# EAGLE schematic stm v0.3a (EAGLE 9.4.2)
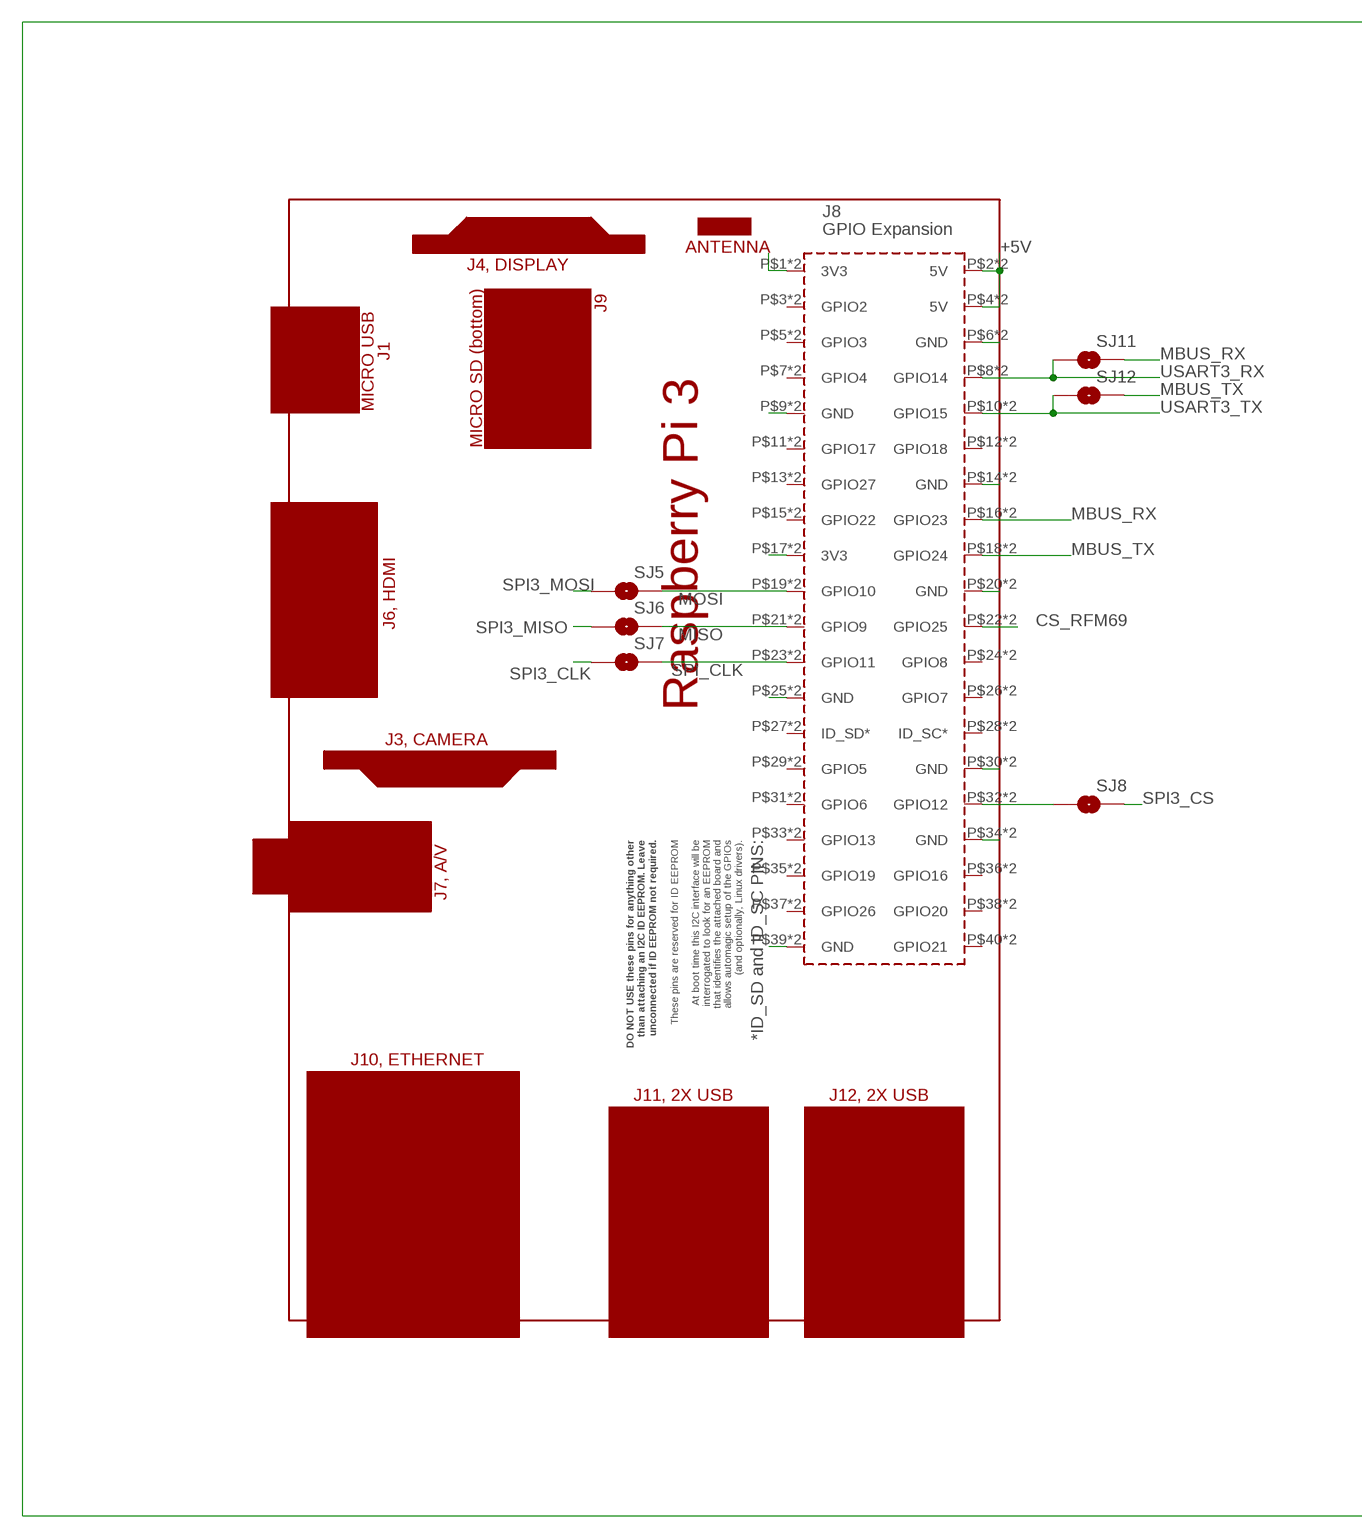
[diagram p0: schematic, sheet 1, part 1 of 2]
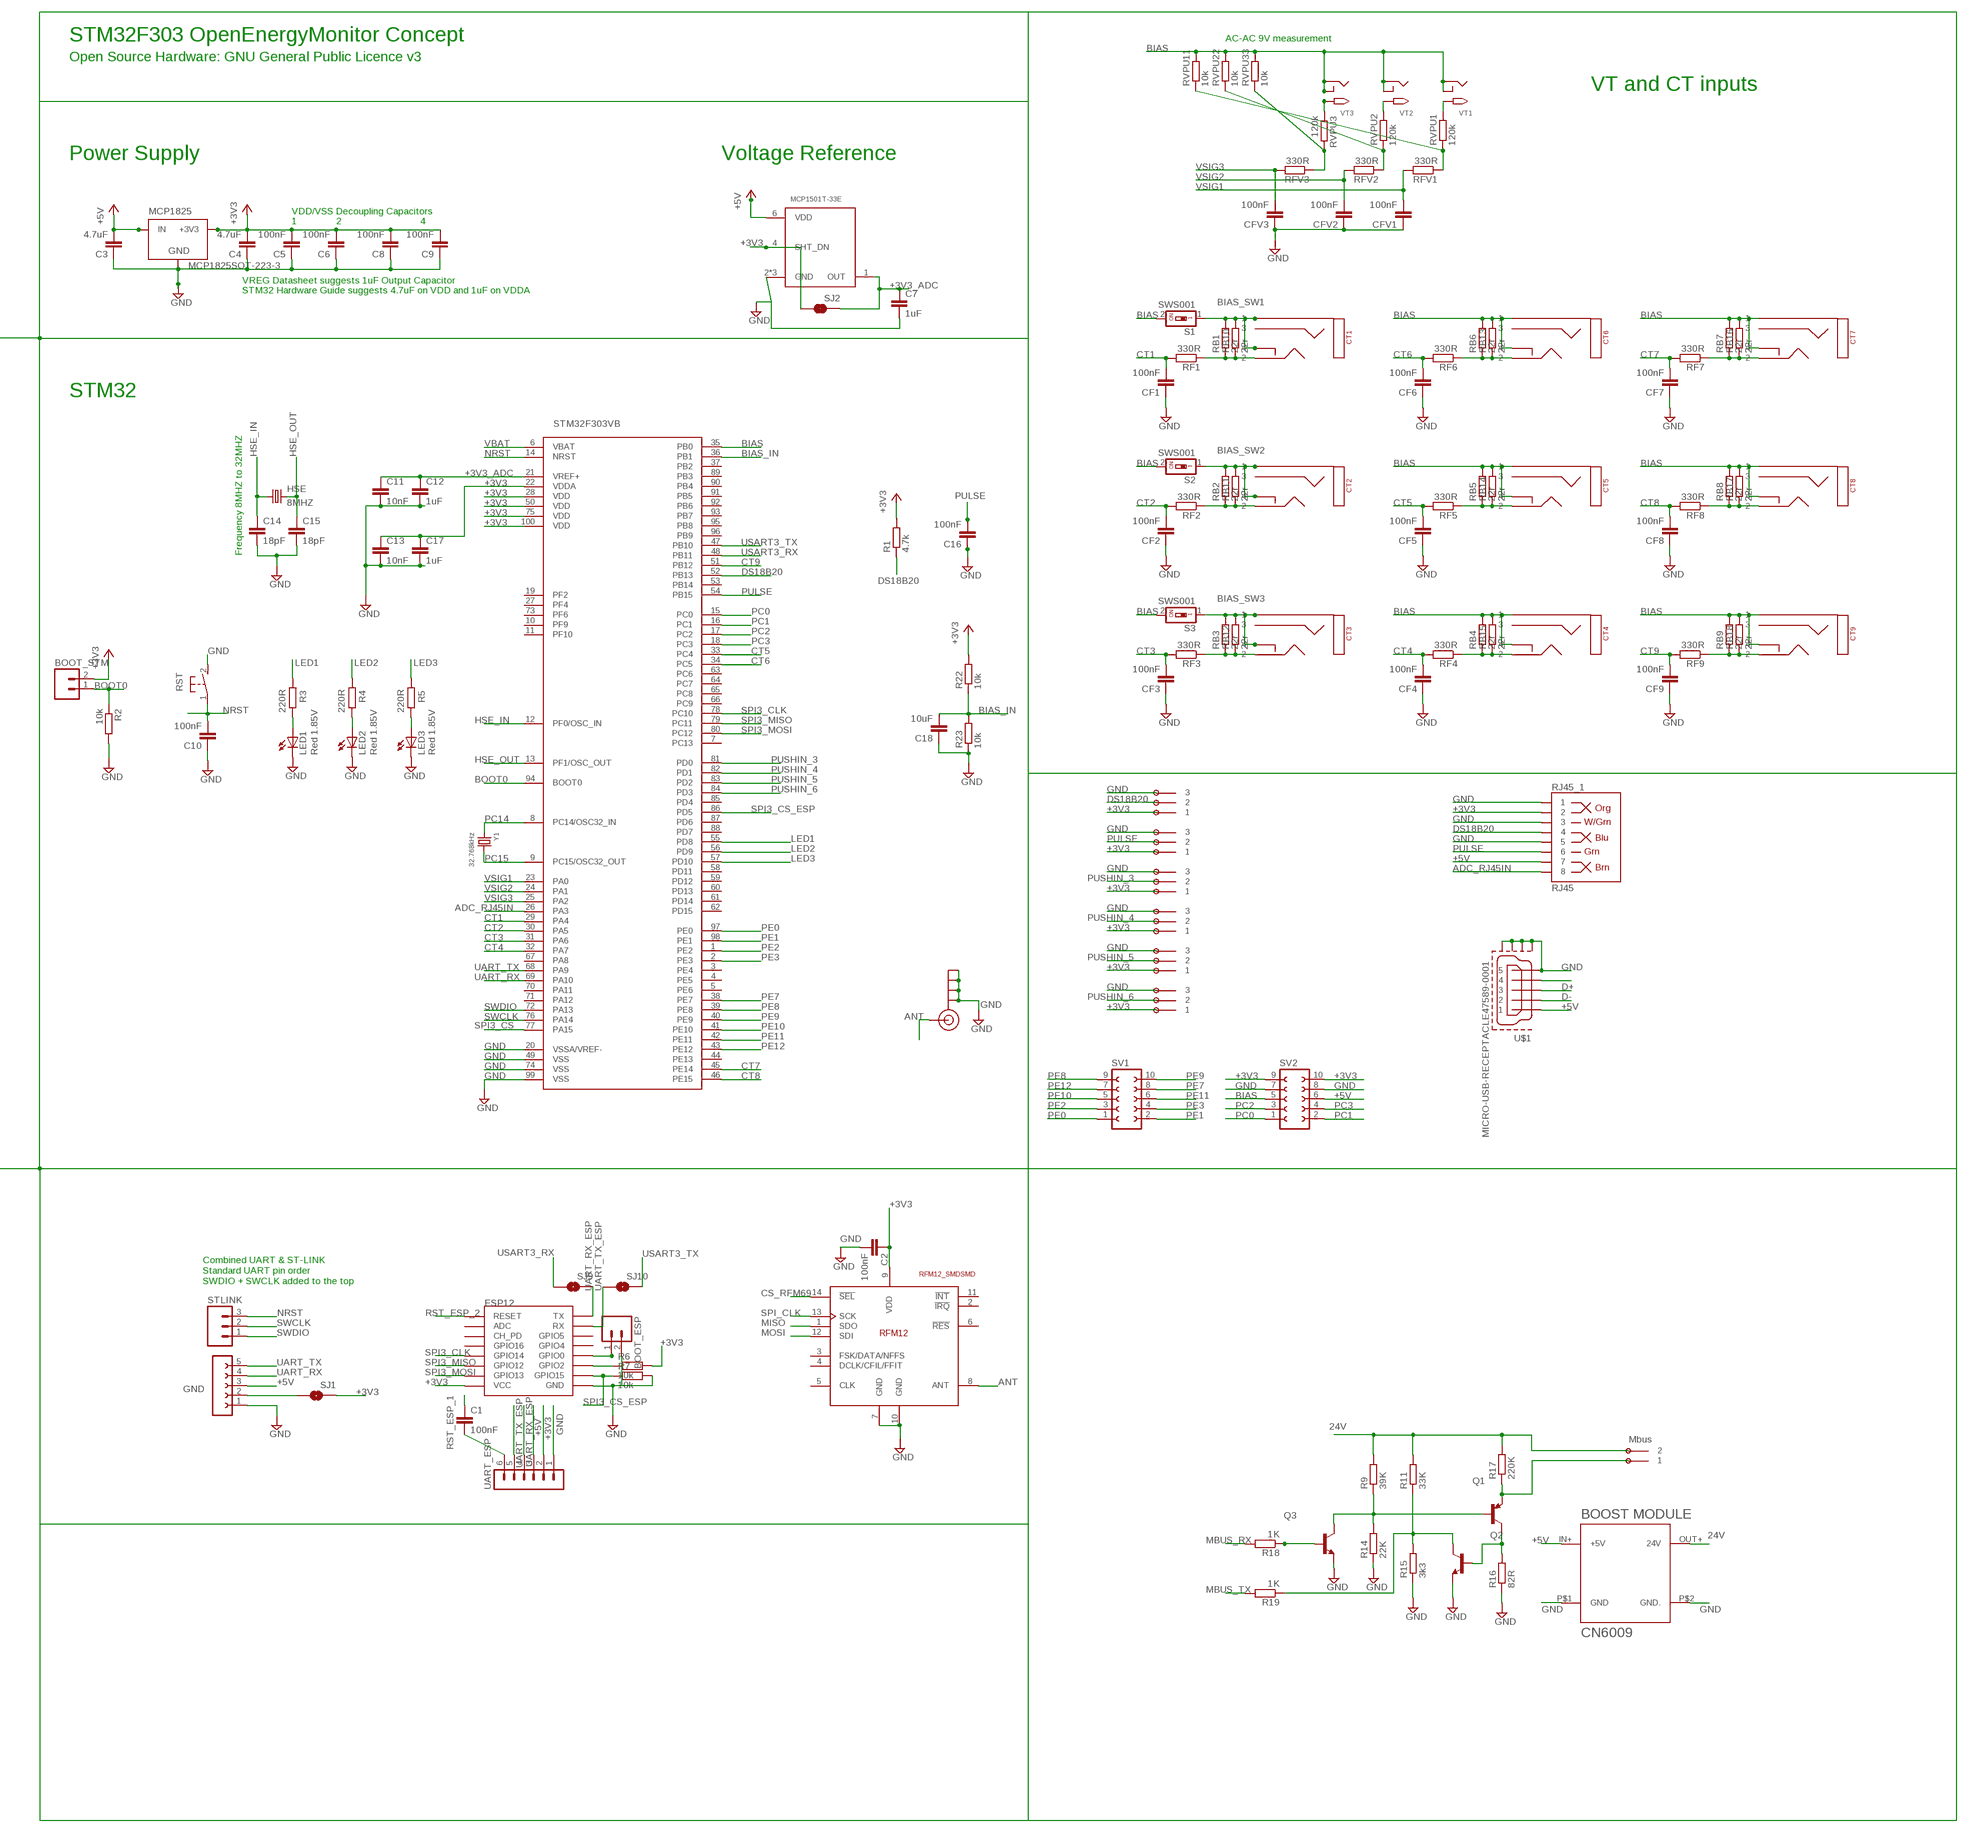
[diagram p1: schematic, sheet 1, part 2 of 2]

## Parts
2POLE_MBUS  OMNIMATE_LSF_2  [OMNIMATE_LSF_2]
3POLE_1  OMNIMATE_LSF_3  [OMNIMATE_LSF_3]
3POLE_2  OMNIMATE_LSF_3  [OMNIMATE_LSF_3]
3POLE_3  OMNIMATE_LSF_3  [OMNIMATE_LSF_3]
3POLE_4  OMNIMATE_LSF_3  [OMNIMATE_LSF_3]
3POLE_5  OMNIMATE_LSF_3  [OMNIMATE_LSF_3]
3POLE_6  OMNIMATE_LSF_3  [OMNIMATE_LSF_3]
BOOT_ESP  M02PTH  [1X02]
BOOT_STM  M02PTH  [1X02]
C1  100nF  C-EUC0603  [C0603]
C2  100nF  C-EUC0603  [C0603]
C3  4.7uF  C-EUC1210  [C1210]
C4  4.7uF  C-EUC0805  [C0805]
C5  100nF  C-EUC0603  [C0603]
C6  100nF  C-EUC0603  [C0603]
C7  1uF  C-EUC0805  [C0805]
C8  100nF  C-EUC0603  [C0603]
C9  100nF  C-EUC0603  [C0603]
C10  100nF  C-EUC0603  [C0603]
C11  10nF  C-EUC0603  [C0603]
C12  1uF  C-EUC0603  [C0603]
C13  10nF  C-EUC0603  [C0603]
C14  18pF  C-EUC0603  [C0603]
C15  18pF  C-EUC0603  [C0603]
C16  100nF  C-EUC0603  [C0603]
C17  1uF  C-EUC0603  [C0603]
C18  10uF  C-EUC0603  [C0603]
CF1  100nF  C-EUC0603  [C0603]
CF2  100nF  C-EUC0603  [C0603]
CF3  100nF  C-EUC0603  [C0603]
CF4  100nF  C-EUC0603  [C0603]
CF5  100nF  C-EUC0603  [C0603]
CF6  100nF  C-EUC0603  [C0603]
CF7  100nF  C-EUC0603  [C0603]
CF8  100nF  C-EUC0603  [C0603]
CF9  100nF  C-EUC0603  [C0603]
CFV1  100nF  C-EUC0603  [C0603]
CFV2  100nF  C-EUC0603  [C0603]
CFV3  100nF  C-EUC0603  [C0603]
CT1  STEREO_SMD  [STEREO_SMT]
CT2  STEREO_SMD  [STEREO_SMT]
CT3  STEREO_SMD  [STEREO_SMT]
CT4  STEREO_SMD  [STEREO_SMT]
CT5  STEREO_SMD  [STEREO_SMT]
CT6  STEREO_SMD  [STEREO_SMT]
CT7  STEREO_SMD  [STEREO_SMT]
CT8  STEREO_SMD  [STEREO_SMT]
CT9  STEREO_SMD  [STEREO_SMT]
ESP12  ESP12SMD  [ESP12-SMD]
GND  UART  FE05-1  [FE05-1]
HSE  8MHZ  CRYSTALCTS406  [CTS406]
J$1  SMA_EDGE  [SMA-EDGE]
LED1  Red 1.85V  LEDCHIP-LED0805  [CHIP-LED0805]
LED2  Red 1.85V  LEDCHIP-LED0805  [CHIP-LED0805]
LED3  Red 1.85V  LEDCHIP-LED0805  [CHIP-LED0805]
MCP1825  MCP1825SOT-223-3  [SOT-223]
PCB2  RPI3YA  [RPI3MIRROR2]
Q1  MMBT3906  [SOT23]
Q2  MMBT3904  [SOT23]
Q3  MMBT3904  [SOT23]
R1  4.7k  R-EU_R0603  [R0603]
R2  10k  R-EU_R0603  [R0603]
R3  220R  R-EU_R0603  [R0603]
R4  220R  R-EU_R0603  [R0603]
R5  220R  R-EU_R0603  [R0603]
R6  10k  R-EU_R0603  [R0603]
R7  10k  R-EU_R0603  [R0603]
R9  39K  R-EU_R0603  [R0603]
R11  33K  R-EU_R0603  [R0603]
R14  22K  R-EU_R0603  [R0603]
R15  3k3  R-EU_R0603  [R0603]
R16  82R  R-EU_R0603  [R0603]
R17  220K  R-EU_R0603  [R0603]
R18  1K  R-EU_R0603  [R0603]
R19  1K  R-EU_R0603  [R0603]
R22  10k  R-EU_R0603  [R0603]
R23  10k  R-EU_R0603  [R0603]
RB1  22r  R-EU_R0603  [R0603]
RB2  22r  R-EU_R0603  [R0603]
RB3  22r  R-EU_R0603  [R0603]
RB4  22r  R-EU_R0603  [R0603]
RB5  22r  R-EU_R0603  [R0603]
RB6  22r  R-EU_R0603  [R0603]
RB7  22r  R-EU_R0603  [R0603]
RB8  22r  R-EU_R0603  [R0603]
RB9  22r  R-EU_R0603  [R0603]
RB10  22r  R-EU_0207/7  [0207/7]
RB11  22r  R-EU_0207/7  [0207/7]
RB12  22r  R-EU_0207/7  [0207/7]
RB13  22r  R-EU_0207/7  [0207/7]
RB14  22r  R-EU_0207/7  [0207/7]
RB15  22r  R-EU_0207/7  [0207/7]
RB16  22r  R-EU_0207/7  [0207/7]
RB17  22r  R-EU_0207/7  [0207/7]
RB18  22r  R-EU_0207/7  [0207/7]
RF1  330R  R-EU_R0603  [R0603]
RF2  330R  R-EU_R0603  [R0603]
RF3  330R  R-EU_R0603  [R0603]
RF4  330R  R-EU_R0603  [R0603]
RF5  330R  R-EU_R0603  [R0603]
RF6  330R  R-EU_R0603  [R0603]
RF7  330R  R-EU_R0603  [R0603]
RF8  330R  R-EU_R0603  [R0603]
RF9  330R  R-EU_R0603  [R0603]
RFM69HCW  RFM12_SMDSMD  [RFM12]
RFV1  330R  R-EU_R0603  [R0603]
RFV2  330R  R-EU_R0603  [R0603]
RFV3  330R  R-EU_R0603  [R0603]
RJ45_1  RJ45  RJ45-8  [RJ45-8]
RST  31-XX  [B3F-31XX]
RVPU1  120k  R-EU_R0603  [R0603]
RVPU2  120k  R-EU_R0603  [R0603]
RVPU3  120k  R-EU_R0603  [R0603]
RVPU11  10k  R-EU_R0603  [R0603]
RVPU22  10k  R-EU_R0603  [R0603]
RVPU33  10k  R-EU_R0603  [R0603]
S1  SWS001  [SMS-001]
S2  SWS001  [SMS-001]
S3  SWS001  [SMS-001]
SJ1  SOLDERJUMPERNO  [SJ_2S-NO]
SJ2  SOLDERJUMPERNO  [SJ_2S-NO]
SJ5  SOLDERJUMPERNO  [SJ_2S-NO]
SJ6  SOLDERJUMPERNO  [SJ_2S-NO]
SJ7  SOLDERJUMPERNO  [SJ_2S-NO]
SJ8  SOLDERJUMPERNO  [SJ_2S-NO]
SJ9  SOLDERJUMPERNO  [SJ_2S-NO]
SJ10  SOLDERJUMPERNO  [SJ_2S-NO]
SJ11  SOLDERJUMPERNO  [SJ_2S-NO]
SJ12  SOLDERJUMPERNO  [SJ_2S-NO]
STLINK  M03PTH  [1X03]
STM32F303VB  STM32F303XB  [TQFP100]
SV1  FE05-2  [FE05-2]
SV2  FE05-2  [FE05-2]
U$1  MICRO-USB-RECEPTACLE47589-0001  [47589-0001]
U$2  BOOST_MODULE  [BOOST]
U$8  MCP1501T-33E  [SOT95P280X145-6N]
UART_ESP  MA06-1  [MA06-1]
VT1  2.1MMJACKSMT  [DCJACK_2MM_SMT]
VT2  2.1MMJACKSMT  [DCJACK_2MM_SMT]
VT3  2.1MMJACKSMT  [DCJACK_2MM_SMT]
Y1  32.768kHz  CRYSTAL8X3.8SMT  [CRYSTAL_8X3.8]

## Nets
24V: 2POLE_MBUS.P$3 2POLE_MBUS.P$4 R9.2 R11.2 R17.2 U$2.OUT+(24V)
+3V3 [power]: 3POLE_1.P$1 3POLE_1.P$2 3POLE_2.P$1 3POLE_2.P$2 3POLE_3.P$1 3POLE_3.P$2 3POLE_4.P$1 3POLE_4.P$2 3POLE_5.P$1 3POLE_5.P$2 3POLE_6.P$1 3POLE_6.P$2 BOOT_STM.2 C2.1 C4.2 C5.2 C6.2 C8.2 C9.2 C13.1 C17.1 ESP12.VCC MCP1825.3(+3V3) R1.2 R6.2 R22.2 RFM69HCW.9(VDD) RJ45_1.2 SJ1.2 SJ2.1 STM32F303VB.22(VDDA) STM32F303VB.28(VDD) STM32F303VB.50(VDD) STM32F303VB.75(VDD) STM32F303VB.100(VDD) SV2.9 SV2.10 U$8.4(SHT_DN) UART_ESP.2
+3V3_ADC: C7.1 C11.1 C12.1 SJ2.2 STM32F303VB.21(VREF+) U$8.1(OUT)
+5V [power]: C3.2 GND.3 MCP1825.1(IN) PCB2.P$2(5V) PCB2.P$4(5V) PCB2.P$42(5V) PCB2.P$44(5V) RJ45_1.7 SV2.6 U$1.1 U$2.IN+(+5V) U$8.6(VDD) UART_ESP.3
AC1: RVPU1.2 VT1.PWR2(TIP)
AC2: RVPU2.2 VT2.PWR2(TIP)
AC3: RVPU3.1 VT3.PWR2(TIP)
ADC0: RFV3.1 RVPU3.2 RVPU33.1
ADC_RJ45IN: RJ45_1.8 STM32F303VB.26(PA3)
ANT: J$1.SIG(SIGNAL) RFM69HCW.8(ANT)
BIAS: CT4.P$1 CT4.P$4 CT5.P$1 CT5.P$4 CT6.P$1 CT6.P$4 CT7.P$1 CT7.P$4 CT8.P$1 CT8.P$4 CT9.P$1 CT9.P$4 RB4.2 RB5.2 RB6.2 RB7.2 RB8.2 RB9.2 RB13.2 RB14.2 RB15.2 RB16.2 RB17.2 RB18.2 RVPU11.2 RVPU22.2 RVPU33.2 S1.2 S2.2 S3.2 STM32F303VB.35(PB0) SV2.5 VT1.GND(RING) VT1.GNDBREAK(RING_SW) VT2.GND(RING) VT2.GNDBREAK(RING_SW) VT3.GND(RING) VT3.GNDBREAK(RING_SW)
BIAS_IN: C18.2 R22.1 R23.2 STM32F303VB.36(PB1)
BIAS_SW1: CT1.P$1 CT1.P$4 RB1.2 RB10.2 S1.1
BIAS_SW2: CT2.P$1 CT2.P$4 RB2.2 RB11.2 S2.1
BIAS_SW3: CT3.P$1 CT3.P$4 RB3.2 RB12.2 S3.1
BOOT0: BOOT_STM.1 R2.1 STM32F303VB.94(BOOT0)
CS_RFM69: PCB2.P$22(GPIO25) PCB2.P$62(GPIO25) RFM69HCW.14(!SEL)
CT1: CF1.2 RF1.2 STM32F303VB.29(PA4)
CT2: CF2.2 RF2.2 STM32F303VB.30(PA5)
CT3: CF3.2 RF3.2 STM32F303VB.31(PA6)
CT4: CF4.2 RF4.2 STM32F303VB.32(PA7)
CT5: CF5.2 RF5.2 STM32F303VB.33(PC4)
CT6: CF6.2 RF6.2 STM32F303VB.34(PC5)
CT7: CF7.2 RF7.2 STM32F303VB.45(PE14)
CT8: CF8.2 RF8.2 STM32F303VB.46(PE15)
CT9: CF9.2 RF9.2 STM32F303VB.51(PB12)
D+: U$1.3
D-: U$1.2
DS18B20: 3POLE_1.P$3 3POLE_1.P$4 R1.1 RJ45_1.4 STM32F303VB.52(PB13)
GND [power]: 3POLE_1.P$5 3POLE_1.P$6 3POLE_2.P$5 3POLE_2.P$6 3POLE_3.P$5 3POLE_3.P$6 3POLE_4.P$5 3POLE_4.P$6 3POLE_5.P$5 3POLE_5.P$6 3POLE_6.P$5 3POLE_6.P$6 BOOT_ESP.2 C2.2 C3.1 C4.1 C5.1 C6.1 C7.2 C8.1 C9.1 C10.1 C11.2 C12.2 C13.2 C14.2 C15.2 C16.1 C17.2 C18.1 CF1.1 CF2.1 CF3.1 CF4.1 CF5.1 CF6.1 CF7.1 CF8.1 CF9.1 CFV1.1 CFV2.1 CFV3.1 ESP12.GND GND.1 J$1.GND@0(GND) J$1.GND@1(GND) J$1.GND@2(GND) J$1.GND@3(GND) LED1.C LED2.C LED3.C MCP1825.2(GND) MCP1825.4(GND) PCB2.P$6(GND) PCB2.P$9(GND) PCB2.P$14(GND) PCB2.P$20(GND) PCB2.P$25(GND) PCB2.P$30(GND) PCB2.P$34(GND) PCB2.P$39(GND) PCB2.P$46(GND) PCB2.P$49(GND) PCB2.P$54(GND) PCB2.P$60(GND) PCB2.P$65(GND) PCB2.P$70(GND) PCB2.P$74(GND) PCB2.P$79(GND) Q2.2(E) Q3.2(E) R2.2 R7.2 R14.1 R15.1 R16.1 R23.1 RFM69HCW.7(GND) RFM69HCW.10(GND) RJ45_1.1 RJ45_1.3 RJ45_1.5 RST.2(S) STM32F303VB.20(VSSA/VREF-) STM32F303VB.49(VSS) STM32F303VB.74(VSS) STM32F303VB.99(VSS) SV2.7 SV2.8 U$1.5 U$1.CASING1(GND1) U$1.CASING2(GND2) U$1.CASING3(GND3) U$1.CASING4(GND4) U$2.P$1(GND) U$2.P$2(GND.) U$8.2(GND) U$8.3(GND) U$8.5(GND) UART_ESP.1
HSE_IN: C14.1 HSE.1 STM32F303VB.12(PF0/OSC_IN)
HSE_OUT: C15.1 HSE.3 STM32F303VB.13(PF1/OSC_OUT)
LED1: R3.2 STM32F303VB.55(PD8)
LED2: R4.2 STM32F303VB.56(PD9)
LED3: R5.2 STM32F303VB.57(PD10)
MBUS_RX: PCB2.P$16(GPIO23) PCB2.P$56(GPIO23) R18.2 SJ11.2
MBUS_TX: PCB2.P$18(GPIO24) PCB2.P$58(GPIO24) R19.2 SJ12.2
MISO: PCB2.P$21(GPIO9) PCB2.P$61(GPIO9) RFM69HCW.1(SDO) SJ6.2
MOSI: PCB2.P$19(GPIO10) PCB2.P$59(GPIO10) RFM69HCW.12(SDI) SJ5.2
N$1: GND.2 SJ1.1
N$2: CT1.P$2 RB1.1 RB10.1 RF1.1
N$5: LED2.A R4.1
N$6: LED3.A R5.1
N$7: BOOT_ESP.1 ESP12.GPIO0
N$8: CT2.P$2 RB2.1 RB11.1 RF2.1
N$10: CT3.P$2 RB3.1 RB12.1 RF3.1
N$11: ESP12.GPIO2 R6.1
N$12: U$1.4
N$16: PCB2.P$32(GPIO12) PCB2.P$72(GPIO12) SJ8.1
N$22: PCB2.P$1(3V3) PCB2.P$41(3V3)
N$24: PCB2.P$17(3V3) PCB2.P$57(3V3)
N$29: 2POLE_MBUS.P$1 2POLE_MBUS.P$2 Q1.2(E) R17.1
N$30: Q1.3(C) Q2.1(B) R16.2
N$31: Q1.1(B) Q3.3(C) R9.1 R14.2
N$32: Q2.3(C) R11.1 R15.2 R19.1
N$33: Q3.1(B) R18.1
N$34: RFV2.1 RVPU2.1 RVPU22.1
N$37: RFV1.1 RVPU1.1 RVPU11.1
N$38: CT4.P$2 RB4.1 RB15.1 RF4.1
N$39: CT5.P$2 RB5.1 RB14.1 RF5.1
N$40: CT6.P$2 RB6.1 RB13.1 RF6.1
N$41: LED1.A R3.1
N$42: CT7.P$2 RB7.1 RB16.1 RF7.1
N$43: CT8.P$2 RB8.1 RB17.1 RF8.1
N$44: CT9.P$2 RB9.1 RB18.1 RF9.1
NRST: C10.2 RST.1(P) STLINK.3 STM32F303VB.14(NRST)
PC0: STM32F303VB.15(PC0) SV2.1
PC1: STM32F303VB.16(PC1) SV2.2
PC2: STM32F303VB.17(PC2) SV2.3
PC3: STM32F303VB.18(PC3) SV2.4
PC14: STM32F303VB.8(PC14/OSC32_IN) Y1.P$1
PC15: STM32F303VB.9(PC15/OSC32_OUT) Y1.P$4
PE0: STM32F303VB.97(PE0) SV1.1
PE1: STM32F303VB.98(PE1) SV1.2
PE2: STM32F303VB.1(PE2) SV1.3
PE3: STM32F303VB.2(PE3) SV1.4
PE7: STM32F303VB.38(PE7) SV1.8
PE8: STM32F303VB.39(PE8) SV1.9
PE9: STM32F303VB.40(PE9) SV1.10
PE10: STM32F303VB.41(PE10) SV1.5
PE11: STM32F303VB.42(PE11) SV1.6
PE12: STM32F303VB.43(PE12) SV1.7
PULSE: 3POLE_2.P$3 3POLE_2.P$4 C16.2 RJ45_1.6 STM32F303VB.54(PB15)
PUSHIN_3: 3POLE_3.P$3 3POLE_3.P$4 STM32F303VB.81(PD0)
PUSHIN_4: 3POLE_4.P$3 3POLE_4.P$4 STM32F303VB.82(PD1)
PUSHIN_5: 3POLE_5.P$3 3POLE_5.P$4 STM32F303VB.83(PD2)
PUSHIN_6: 3POLE_6.P$3 3POLE_6.P$4 STM32F303VB.84(PD3)
RST_ESP_1: C1.2 UART_ESP.6
RST_ESP_2: C1.1 ESP12.RESET
SPI3_CLK: ESP12.GPIO14 SJ7.1 STM32F303VB.78(PC10)
SPI3_CS: SJ8.2 STM32F303VB.77(PA15)
SPI3_CS_ESP: ESP12.GPIO15 R7.1 STM32F303VB.86(PD5)
SPI3_MISO: ESP12.GPIO12 SJ6.1 STM32F303VB.79(PC11)
SPI3_MOSI: ESP12.GPIO13 SJ5.1 STM32F303VB.80(PC12)
SPI_CLK: PCB2.P$23(GPIO11) PCB2.P$63(GPIO11) RFM69HCW.13(SCK) SJ7.2
SWCLK: STLINK.2 STM32F303VB.76(PA14)
SWDIO: STLINK.1 STM32F303VB.72(PA13)
UART_RX: GND.4 STM32F303VB.69(PA10)
UART_RX_ESP: ESP12.TXD0(TX) SJ9.2 UART_ESP.4
UART_TX: GND.5 STM32F303VB.68(PA9)
UART_TX_ESP: ESP12.RXD0(RX) SJ10.1 UART_ESP.5
USART3_RX: PCB2.P$8(GPIO14) PCB2.P$48(GPIO14) SJ9.1 SJ11.1 STM32F303VB.48(PB11)
USART3_TX: PCB2.P$10(GPIO15) PCB2.P$50(GPIO15) SJ10.2 SJ12.1 STM32F303VB.47(PB10)
VBAT: STM32F303VB.6(VBAT)
VSIG1: CFV1.2 RFV1.2 STM32F303VB.23(PA0)
VSIG2: CFV2.2 RFV2.2 STM32F303VB.24(PA1)
VSIG3: CFV3.2 RFV3.2 STM32F303VB.25(PA2)
Unconnected: CT1.P$3 CT2.P$3 CT3.P$3 CT4.P$3 CT5.P$3 CT6.P$3 CT7.P$3 CT8.P$3 CT9.P$3 ESP12.ADC ESP12.CH_PD ESP12.GPIO4 ESP12.GPIO5 ESP12.GPIO16 PCB2.P$3(GPIO2) PCB2.P$5(GPIO3) PCB2.P$7(GPIO4) PCB2.P$11(GPIO17) PCB2.P$12(GPIO18) PCB2.P$13(GPIO27) PCB2.P$15(GPIO22) PCB2.P$24(GPIO8) PCB2.P$26(GPIO7) PCB2.P$27(ID_SD*) PCB2.P$28(ID_SC*) PCB2.P$29(GPIO5) PCB2.P$31(GPIO6) PCB2.P$33(GPIO13) PCB2.P$35(GPIO19) PCB2.P$36(GPIO16) PCB2.P$37(GPIO26) PCB2.P$38(GPIO20) PCB2.P$40(GPIO21) PCB2.P$43(GPIO2) PCB2.P$45(GPIO3) PCB2.P$47(GPIO4) PCB2.P$51(GPIO17) PCB2.P$52(GPIO18) PCB2.P$53(GPIO27) PCB2.P$55(GPIO22) PCB2.P$64(GPIO8) PCB2.P$66(GPIO7) PCB2.P$67(ID_SD*) PCB2.P$68(ID_SC*) PCB2.P$69(GPIO5) PCB2.P$71(GPIO6) PCB2.P$73(GPIO13) PCB2.P$75(GPIO19) PCB2.P$76(GPIO16) PCB2.P$77(GPIO26) PCB2.P$78(GPIO20) PCB2.P$80(GPIO21) RFM69HCW.2(!IRQ) RFM69HCW.3(FSK/DATA/NFFS) RFM69HCW.4(DCLK/CFIL/FFIT) RFM69HCW.5(CLK) RFM69HCW.6(!RES) RFM69HCW.11(!INT) STM32F303VB.3(PE4) STM32F303VB.4(PE5) STM32F303VB.5(PE6) STM32F303VB.7(PC13) STM32F303VB.10(PF9) STM32F303VB.11(PF10) STM32F303VB.19(PF2) STM32F303VB.27(PF4) STM32F303VB.37(PB2) STM32F303VB.44(PE13) STM32F303VB.53(PB14) STM32F303VB.58(PD11) STM32F303VB.59(PD12) STM32F303VB.60(PD13) STM32F303VB.61(PD14) STM32F303VB.62(PD15) STM32F303VB.63(PC6) STM32F303VB.64(PC7) STM32F303VB.65(PC8) STM32F303VB.66(PC9) STM32F303VB.67(PA8) STM32F303VB.70(PA11) STM32F303VB.71(PA12) STM32F303VB.73(PF6) STM32F303VB.85(PD4) STM32F303VB.87(PD6) STM32F303VB.88(PD7) STM32F303VB.89(PB3) STM32F303VB.90(PB4) STM32F303VB.91(PB5) STM32F303VB.92(PB6) STM32F303VB.93(PB7) STM32F303VB.95(PB8) STM32F303VB.96(PB9)

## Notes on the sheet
- STM32F303 OpenEnergyMonitor Concept | AC-AC 9V measurement
- Open Source Hardware: GNU General Public Licence v3
- VT and CT inputs
- Power Supply | Voltage Reference
- VDD/VSS Decoupling Capacitors
- 1 | 2 | 4
- VREG Datasheet suggests 1uF Output Capacitor
- STM32 Hardware Guide suggests 4.7uF on VDD and 1uF on VDDA
- STM32
- Frequency 8MHZ to 32MHZ
- Combined UART & ST-LINK
  Standard UART pin order
  SWDIO + SWCLK added to the top
- Mbus

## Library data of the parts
2POLE_MBUS = OMNIMATE_LSF:OMNIMATE_LSF_2
3POLE_1-3POLE_6 = OMNIMATE_LSF:OMNIMATE_LSF_3
BOOT_ESP BOOT_STM = SparkFun:M02: Header 2
C1 C2 C5 C6 C8-C18 CF1-CF9 CFV1-CFV3 = resistor:C-EU: CAPACITOR, European symbol
C3 C4 C7 = rcl:C-EU: CAPACITOR, European symbol; SPICEPREFIX: C
CT1-CT9 = IotaWatt_parts:STEREO_SMD: 3.5mm Stereo Jack SMT
ESP12 = ESP8266 MODULES _ CORRECTED:ESP12: ESP8266 Wifi module 12
GND = con-lsta:FE05-1: FEMALE HEADER; OC_FARNELL: unknown; OC_NEWARK: unknown
HSE = crystal:CRYSTAL: CRYSTAL; OC_FARNELL: unknown; OC_NEWARK: unknown
J$1 = SparkFun-Connectors:SMA_EDGE: SMA Antenna Connector End launch SMA connector. The paste layer has been removed so that the connector can be hand soldered onto the board after reflow.
LED1-LED3 = adafruit:LED: LED
MCP1825 = SteelCaveRobotics-Power:MCP1825: MCP1825 3.3v LDO Linear Regulator
PCB2 = e14_Rpi3_RevA+mirror-pcb copy:RPI3: Device for Raspberry Pi 3 board created by Dave Young for www.element14.com More information and support community is available at https://www.element14.com/community/community/raspberry-pi Device for Raspberry Pi 3 board updated by Gerald Schwarz for www.element14.com On RPI3 addet the layer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
Q1 = Transistor:MMBT3906: TRANS PNP 40V 0.2A SOT-23; CREATED_BY: PCB Layout; DIGIKEY_PART_NUMBER: MMBT3906FSCT-ND; MANUFACTURER: ON Semiconductor; MPN: MMBT3906; PACKAGE: SOT-23
Q2 Q3 = Transistor:MMBT3904: TRANS NPN 40V 0.2A SOT-23; CREATED_BY: PCB Layout; DIGIKEY_PART_NUMBER: MMBT3904FSCT-ND; MANUFACTURER: ON Semiconductor; MPN: MMBT3904; PACKAGE: SOT-23-3
R1 R2 R6 R7 R22 R23 RB1-RB9 RF1-RF9 RFV1-RFV3 RVPU1-RVPU3 RVPU11 RVPU22 RVPU33 = resistor:R-EU_: RESISTOR, European symbol
R3-R5 R9 R11 R14-R19 RB10-RB18 = rcl:R-EU_: RESISTOR, European symbol; SPICEPREFIX: R
RFM69HCW = rfm12b _ rfm69cw:RFM12_SMD: RFM12 is a low costing ISM band transceiver module implemented with unique PLL. It works signal ranges from 315/433/868/915MHZ bands, comply with FCC, ETSI regulation. The SPI interface is used to communicate with microcontroller for parameter setting.
RJ45_1 = SparkFun-Connectors:RJ45-8: RJ45 Jack - 8 pin Simple RJ45, 8-pin connection. Commonly used for Cat5, Cat5e, and Cat6 Ethernet cables. Here is the connector we sell at SparkFun: RJ45 8-Pin Connector (PRT-00643) Datasheet It is used on this SparkFun product: SparkFun RJ45 Breakout (BOB-00716) Note, you may also be interested in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; PROD_ID: CONN-08506; SF_ID: PRT-00643
RST = switch-omron:31-XX: OMRON SWITCH; MPN: B3F-3100; OC_FARNELL: 959704; OC_NEWARK: 36M3582
S1-S3 = smd-special:SWS001: SMD Dip Switch 1 pol.
SJ1 SJ2 SJ5-SJ12 = SparkFun:SOLDERJUMPER: Solder Jumper
STLINK = SparkFun:M03: Header 3 Standard 3-pin 0.1" header. Use with straight break away headers (SKU : PRT-00116), right angle break away headers (PRT-00553), swiss pins (PRT-00743), machine pins (PRT-00117), and female headers (PRT-00115). Molex polarized connector foot print use with SKU : PRT-08232 with associated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
STM32F303VB = stm32f303:STM32F303XB
SV1 SV2 = con-lsta-RFM69Pi:FE05-2: FEMALE HEADER; OC_FARNELL: unknown; OC_NEWARK: unknown
U$1 = con-molex-usb:MICRO-USB-RECEPTACLE: MICRO USB RECEPTACLES Micro-USB Receptacles, SMT, Lead-Free from MOLEX. (C) 2014 Tomasz Boleslaw CEDRO, cederom@tlen.pl, http://www.tomek.cedro.info. Version 0.1 (2014-01-17): Initial release. Version 0.2 (2014-02-06): Updated 47589-0001 footprint pins/pads/milling. Following devices are included: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
U$2 = BOOST MODULE CN6009:BOOST_MODULE
U$8 = MCP1501T-33E:MCP1501T-33E
UART_ESP = con-lstb-db:MA06-1: PIN HEADER; OC_FARNELL: unknown; OC_NEWARK: unknown
VT1-VT3 = adafruit:2.1MMJACK: 2.1mm x 5.5mm THM DC jack with internal switch. Digikey part #PJ-102A, 4UCON part #05537 2.1mm x 5.5mm SMT DC jack with internal switch. Digikey part #PJ-002A-SMT, 4UCON part #03267 By microbuilder.eu & adafruit.com
Y1 = microbuilder:CRYSTAL: Crystals

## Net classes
0 default: width 0.203 mm, drill 0.35 mm, clearance 0.152 mm
1 power: width 0.279 mm, drill 0.35 mm, clearance 0.178 mm
2 gnd: width 0.254 mm, drill 0.35 mm, clearance 0.152 mm

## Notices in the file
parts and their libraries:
SparkFun-Connectors: Licensing: Creative Commons ShareAlike 4.0 International - https://creativecommons.org/licenses/by-sa/4.0
microbuilder: This work is placed in the public domain, and may be freely used for commercial and non-commercial work with the following conditions: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
